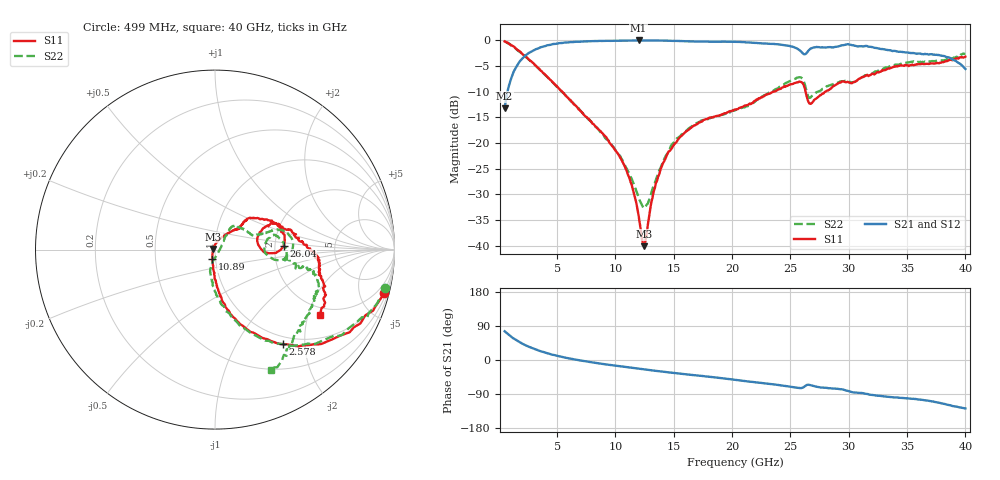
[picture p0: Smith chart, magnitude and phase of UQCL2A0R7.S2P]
! AVX Corporation
! Date:  10/27/06
! Part No:  UQCL2A0R7
! Description:  Ultra Low ESR Microwave capacitors
! Mounting Orientation:  Horizontal
# GHZ S DB R 50
! Freq  |S11|  S11 Ph  |S21|  S21 Ph  |S12|  S12 Ph  |S22|  S22 Ph
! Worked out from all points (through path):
!   400 points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, 499 MHz to 40 GHz, reference 50 ohm
!   highest |S21| = -0.05 dB at 11.98 GHz (marker M1); lowest = -13.3 dB at 499 MHz (marker M2)
!   group delay of S21, straight-line fit = 11 ps
!   lowest |S11| = -40.1 dB at 12.48 GHz (marker M3), VSWR 1.02, Z = 49.1 + j0.344 ohm
!   |S11| at or under -10 dB: 5.426 GHz to 23.6 GHz (18.17 GHz wide, 125 % of centre); 26.3 GHz to 28.01 GHz (1.714 GHz wide, 6.31 % of centre)
!   |S22| runs from -32.7 to -0.3 dB; largest |S21 - S12| = 0.012
!   S11 on the Smith chart (normalised r, x): 499 MHz: 0.84, -7.84; 2.578 GHz: 0.87, -1.59; 10.89 GHz: 0.97, -0.10; 26.04 GHz: 2.23, +0.10; 40 GHz: 1.71, -2.40
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0.499  -0.23 -14.4  -13.26 75.8  -13.26 76.1  -0.27 -12.9
1.291  -1.25 -32.7  -6.05 56.5  -6.09 55.6  -1.38 -33.8
2.578  -3.75 -54.2  -2.48 34.9  -2.54 35.1  -3.78 -54.4
4.558  -8.01 -74.0  -0.82 14.2  -0.82 14.3  -8.06 -76.1
7.132  -14.01 -87.3  -0.26 -1.8  -0.32 -1.9  -14.08 -94.0
10.894  -25.08 -105.5  -0.09 -18.6  -0.08 -18.5  -24.72 -97.6
11.983  -34.05 -131.4  -0.05 -22.9  -0.06 -22.9  -30.53 -66.9
12.478  -40.06 159.3  -0.05 -24.8  -0.06 -24.9  -32.68 -27.9
13.072  -31.55 90.9  -0.06 -27.1  -0.06 -27.1  -29.76 17.0
13.666  -26.49 73.3  -0.06 -29.3  -0.07 -29.4  -25.86 37.3
14.557  -21.64 59.8  -0.10 -32.7  -0.11 -32.6  -21.65 49.9
16.042  -17.77 49.9  -0.20 -37.8  -0.21 -37.6  -17.66 53.7
20.299  -13.47 43.4  -0.32 -52.5  -0.33 -52.2  -13.58 27.0
24.457  -8.97 27.2  -0.93 -68.2  -0.96 -67.9  -8.60 17.0
26.041  -8.34 3.0  -2.51 -73.1  -2.44 -72.5  -7.51 -2.9
26.536  -11.97 2.1  -2.06 -65.3  -2.03 -65.5  -11.07 -3.9
26.833  -12.23 15.6  -1.55 -67.0  -1.52 -67.5  -10.86 8.1
27.922  -10.11 24.5  -1.40 -73.2  -1.35 -73.3  -9.17 13.4
29.902  -8.08 14.5  -0.77 -81.3  -0.79 -81.2  -8.05 -6.5
33.466  -5.52 0.5  -1.94 -97.5  -1.96 -97.3  -5.13 -12.9
37.228  -4.52 -10.5  -2.82 -109.3  -2.74 -108.6  -4.07 -30.1
40  -3.20 -32.0  -5.59 -127.9  -5.63 -127.8  -2.62 -65.2
